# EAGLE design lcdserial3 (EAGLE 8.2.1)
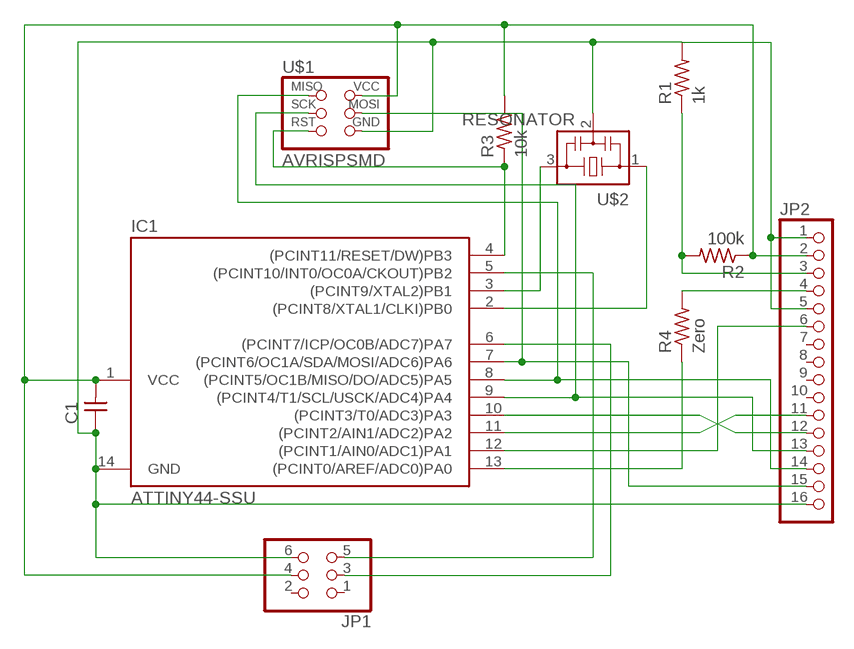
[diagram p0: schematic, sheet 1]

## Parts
C1  CAP-UNPOLARIZEDFAB  [C1206FAB]
IC1  ATTINY44-SSU  [SOIC14]
JP1  PINHD-2X3-SMD  [2X03SMD]
JP2  PINHD-1X16  [1X16]
R1  1k  RES-US1206FAB  [R1206FAB]
R2  100k  RES-US1206FAB  [R1206FAB]
R3  10k  RES-US1206FAB  [R1206FAB]
R4  Zero  RES-US1206FAB  [R1206FAB]
U$1  AVRISPSMD  [2X03SMD]
U$2  RESONATOR  [EFOBM]

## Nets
N$1: IC1.3((PCINT9/XTAL2)PB1) U$2.3
N$2: IC1.2((PCINT8/XTAL1/CLKI)PB0) U$2.1
N$3: C1.1 IC1.14(GND) JP1.6 JP2.1 JP2.5 JP2.16 R1.2 U$1.6(GND) U$2.2
N$4: IC1.6((PCINT7/ICP/OC0B/ADC7)PA7) JP1.3
N$5: JP2.4 R4.2
N$6: JP2.3 R1.1 R2.2
N$7: IC1.10((PCINT3/T0/ADC3)PA3) JP2.12
N$8: IC1.9((PCINT4/T1/SCL/USCK/ADC4)PA4) JP2.13 U$1.3(SCK)
N$9: IC1.4((PCINT11/RESET/DW)PB3) R3.1 U$1.5(RST)
N$10: IC1.11((PCINT2/AIN1/ADC2)PA2) JP2.11
N$11: IC1.12((PCINT1/AIN0/ADC1)PA1) JP2.6
N$12: IC1.13((PCINT0/AREF/ADC0)PA0) R4.1
N$14: IC1.8((PCINT5/OC1B/MISO/DO/ADC5)PA5) JP2.14 U$1.1(MISO)
N$15: C1.2 IC1.1(VCC) JP1.4 JP2.2 R2.1 R3.2 U$1.2(VCC)
N$16: IC1.7((PCINT6/OC1A/SDA/MOSI/ADC6)PA6) JP2.15 U$1.4(MOSI)
N$20: IC1.5((PCINT10/INT0/OC0A/CKOUT)PB2) JP1.5
Unconnected: JP1.1 JP1.2 JP2.7 JP2.8 JP2.9 JP2.10

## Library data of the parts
C1 = fab:CAP-UNPOLARIZED
IC1 = fab:ATTINY44
JP1 = fab:PINHD-2X3-SMD: PIN HEADER
JP2 = pinhead:PINHD-1X16: PIN HEADER
R1-R4 = fab:RES-US: Resistor (US Symbol)
U$1 = fab:AVRISP
U$2 = fab:RESONATOR

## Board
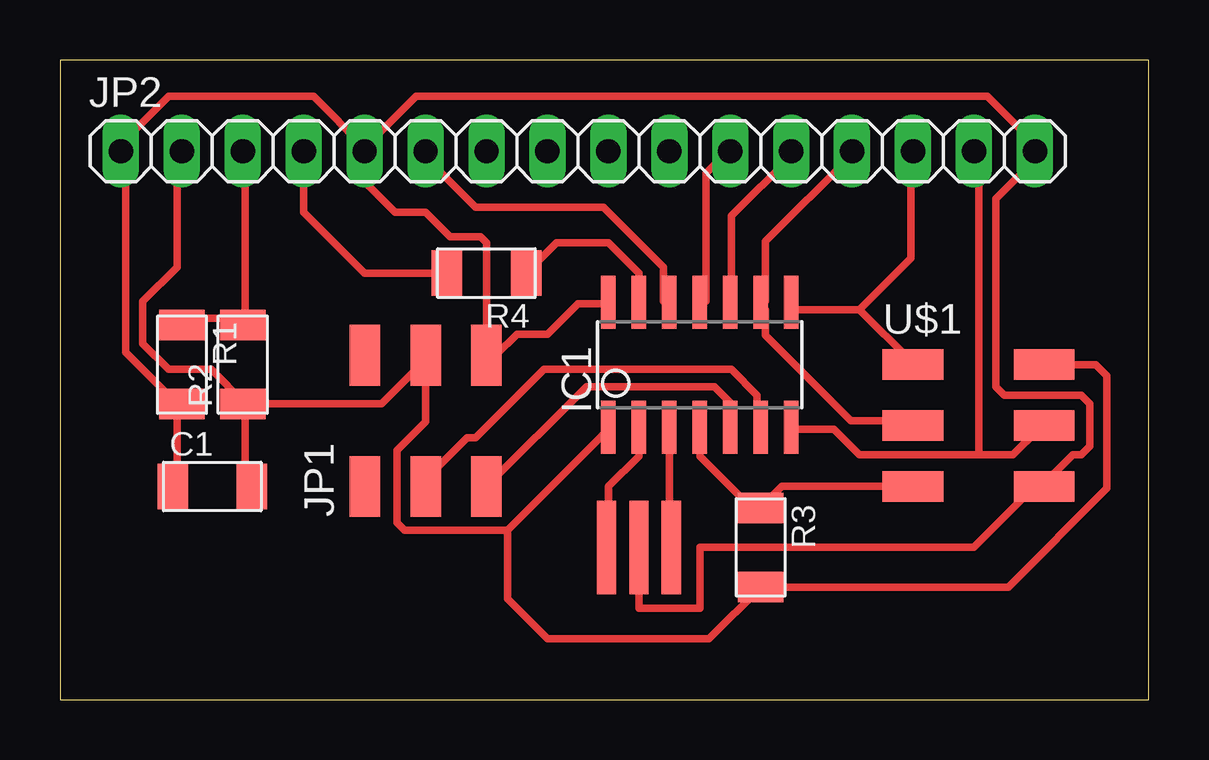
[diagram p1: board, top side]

Size 45.39 x 26.66 mm. Coordinates in mm from the lower left corner, seen from the top.
Outline: 0,0 45.39,0 45.39,26.66 0,26.66 0,0
Copper layers (1*16): Top 0.035mm / dielectric 1.5mm / Bottom 0.035mm
Design rules "default *": minimum track width 12mil, minimum drill 0.35mm, track to track 16mil, track to pad 16mil, pad to pad 16mil, via to via 16mil, smd to smd 16mil, copper to edge 40mil, drill to drill 6mil, minimum pad ring 10mil, minimum via ring 8mil, stop-mask expansion 4mil, vias tented up to drill 0mil, thermal gap 10mil

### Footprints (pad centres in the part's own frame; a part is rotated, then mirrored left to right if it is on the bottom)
C1206FAB = smd 1.27 x 1.905: 1 -1.651,0; 2 1.651,0
SOIC14 = smd 0.61 x 2.21: 1 -3.81,-2.603; 2 -2.54,-2.603; 3 -1.27,-2.603; 4 0,-2.603; 5 1.27,-2.603; 6 2.54,-2.603; 7 3.81,-2.603; 8 3.81,2.603; 9 2.54,2.603; 10 1.27,2.603; 11 0,2.603; 12 -1.27,2.603; 13 -2.54,2.603; 14 -3.81,2.603
2X03SMD = smd 2.54 x 1.27: 1 -2.54,2.54; 2 2.92,2.54; 3 -2.54,0; 4 2.92,0; 5 -2.54,-2.54; 6 2.92,-2.54
1X16 = drill 1.016 long: 1 -19.05,0; 2 -16.51,0; 3 -13.97,0; 4 -11.43,0; 5 -8.89,0; 6 -6.35,0; 7 -3.81,0; 8 -1.27,0; 9 1.27,0; 10 3.81,0; 11 6.35,0; 12 8.89,0; 13 11.43,0; 14 13.97,0; 15 16.51,0; 16 19.05,0
R1206FAB = smd 1.27 x 1.905: 1 -1.651,0; 2 1.651,0
EFOBM = smd 0.8 x 3.9: 1 -1.35,0; 2 0,0; 3 1.35,0

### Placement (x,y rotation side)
C1  6.35,8.89 0 top
IC1  26.67,13.97 0 top
JP1  15.24,11.43 90 top
JP2  21.59,22.86 0 top
R1  5.08,13.97 270 top
R2  7.62,13.97 90 top
R3  29.21,6.35 270 top
R4  17.78,17.78 180 top
U$1  38.1,11.43 0 top
U$2  24.13,6.35 0 top

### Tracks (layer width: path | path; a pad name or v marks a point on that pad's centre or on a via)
N$1
  Top 0.305: IC1.3 25.4,6.43 U$2.3
N$2
  Top 0.305: IC1.2 24.13,10.16 22.86,8.89 22.86,6.43 U$2.1
N$3
  Top 0.305: C1.1 4.88,9.14 4.88,11.99 R1.2 4.88,12.34 2.74,14.48 2.74,22.66 JP2.1 2.39,23.01 4.52,25.15 10.57,25.15 12.7,23.01 | 12.7,23.01 14.83,25.15 38.66,25.15 40.79,23.01 JP2.16 40.79,22.66 39.01,20.88 39.01,13.06 39.37,12.7 42.57,12.7 42.93,12.34 42.93,10.57 42.57,10.21 42.22,10.21 41.15,9.14 U$1.6 40.64,8.89 38.1,6.35 26.67,6.35 26.67,3.81 24.13,3.81 U$2.2 | 12.7,23.01 JP2.5 12.7,21.59 13.97,20.32 15.24,20.32 16.27,19.29 17.54,19.29 17.78,19.05 JP1.6 | JP1.6 17.78,13.97 | JP1.6 18.16,14.35 19.05,15.24 20.32,15.24 21.59,16.51 22.8,16.51 IC1.14
N$4
  Top 0.305: IC1.6 29.06,11.63 29.06,12.7 27.99,13.77 20.17,13.77 17.32,10.92 16.97,10.92 15.19,9.14 JP1.3
N$5
  Top 0.305: R4.2 12.7,17.78 10.16,20.32 JP2.4
N$6
  Top 0.305: R1.1 5.23,15.9 7.37,15.9 R2.2 7.72,15.9 7.72,22.66 JP2.3
N$7
  Top 0.305: IC1.10 27.99,16.61 27.99,20.17 30.48,22.66 JP2.12
N$8
  Top 0.305: JP2.13 32.97,22.66 29.41,19.1 29.41,16.61 IC1.9 29.41,16.26 29.41,15.19 32.97,11.63 35.46,11.63 U$1.3
N$9
  Top 0.305: U$1.5 30.1,8.89 R3.1 28.83,8 26.67,10.16 IC1.4
N$10
  Top 0.305: IC1.11 26.92,16.61 26.92,21.95 27.64,22.66 JP2.11
N$11
  Top 0.305: IC1.12 25.15,16.61 25.15,18.03 22.66,20.52 17.32,20.52 15.19,22.66 JP2.6
N$12
  Top 0.305: IC1.13 24.13,17.78 22.86,19.05 20.7,19.05 R4.1
N$14
  Top 0.305: 33.33,16.26 30.48,16.26 IC1.8 | 33.33,16.26 35.46,14.12 U$1.1 | 33.33,16.26 35.46,18.39 35.46,22.66 JP2.14
N$15
  Top 0.305: C1.2 7.72,9.14 7.72,11.99 R2.1 7.72,12.34 | 7.72,12.34 13.41,12.34 15.19,14.12 JP1.4 15.24,11.59 14.05,10.39 14.05,7.39 14.37,7.06 18.65,7.06 | 7.72,12.34 6.3,13.77 4.52,13.77 3.45,14.83 3.45,16.61 4.88,18.03 4.88,22.66 JP2.2 | IC1.1 22.86,11.28 18.65,7.06 | 18.65,7.06 18.65,4.21 20.32,2.54 27.05,2.54 R3.2 39.52,4.7 43.64,8.81 43.64,13.51 43.18,13.97 U$1.2
N$16
  Top 0.305: 38.3,10.21 39.73,10.21 40.79,11.28 U$1.4 | 38.3,10.21 33.33,10.21 32.26,11.28 30.48,11.28 IC1.7 | 38.3,10.21 38.3,22.66 JP2.15
N$20
  Top 0.305: JP1.5 21.95,13.06 27.28,13.06 27.99,12.34 27.99,11.63 IC1.5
